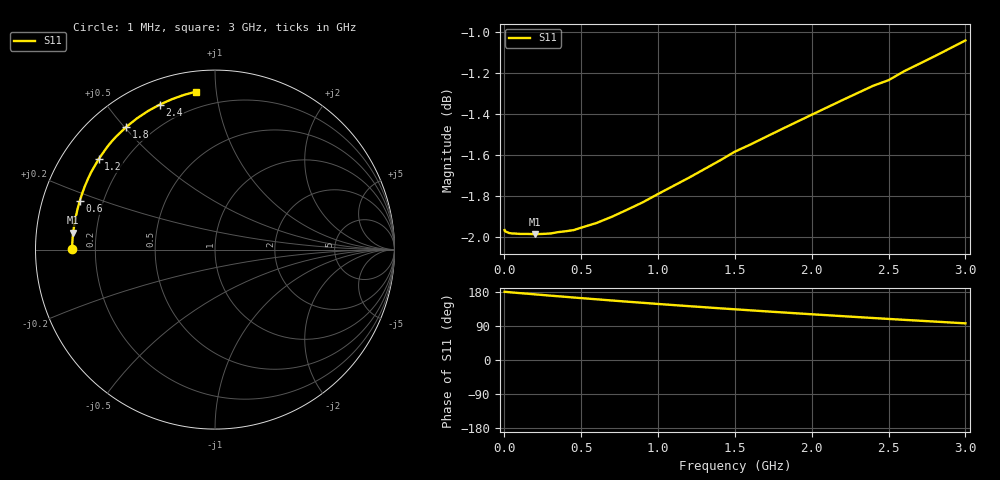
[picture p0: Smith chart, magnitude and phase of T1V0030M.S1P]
! SIEMENS Small Signal Semiconductors
! BAT68-04
! Si Schottky Diode (2 diodes in series, pin 3 open) in SOT23
! IF = 30 mA
! S-Parameters:  August  1994
# GHz  S  MA  R  50
!  f  S11
! GHz  MAG  ANG
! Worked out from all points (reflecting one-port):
!   33 points, 1 MHz to 3 GHz, reference 50 ohm
!   lowest |S11| = -2.0 dB at 200 MHz (marker M1), VSWR 8.79, Z = 5.71 + j2.93 ohm
!   phase of S11 starts at 180 deg and turns -83 deg over the sweep
!   S11 on the Smith chart (normalised r, x): 1 MHz: 0.11, +0.00; 600 MHz: 0.11, +0.17; 1.2 GHz: 0.11, +0.34; 1.8 GHz: 0.11, +0.51; 2.4 GHz: 0.11, +0.68; 3 GHz: 0.11, +0.88
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0.001  0.7975 179.9
0.003  0.797 179.8
0.01  0.7968 179.7
0.1  0.7958 176.5
0.15  0.7958 174.9
0.2  0.7957 173.2
0.3  0.796 169.8
0.35  0.7966 168.2
0.4  0.797 166.6
0.45  0.7975 164.9
0.5  0.7986 163.3
0.6  0.8007 160.2
0.7  0.8035 157.0
0.8  0.8067 153.9
0.9  0.81 150.9
1  0.8138 147.9
1.2  0.8212 142.1
1.4  0.8291 136.5
1.5  0.8333 133.8
1.6  0.8366 131.1
1.8  0.8437 125.8
2  0.8507 120.7
2.2  0.8577 115.7
2.4  0.8646 110.8
2.5  0.8673 108.4
2.6  0.8716 106.0
2.8  0.879 101.4
3  0.8868 96.7
